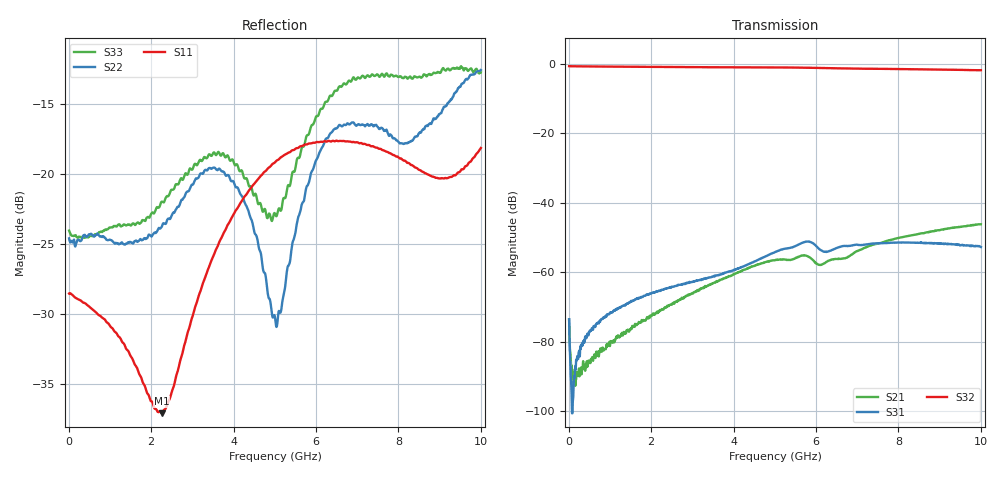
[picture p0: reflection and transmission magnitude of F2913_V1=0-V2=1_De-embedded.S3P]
! Webpage:  http://www.idt.com/
! Timing and RF Division
! 515 Groton Road, Suite 102
! Westford, MA 01886-6024
! Device:  F2913
! Description: High Isolation SP2T RF Switch
! Frequency:  0.050 -  6.000 GHz
! Package:  4x4 mm QFN Plastic Package: 20 pin
! Ports:  3 RF, 3 DC
!  Pin  1  = GND
!  Pin  2  = GND
!  Pin  3  = RF1  =  Port 1
!  Pin  4  = GND
!  Pin  5  = GND
!  Pin  6  = GND
!  Pin  7  = GND
!  Pin  8  = RFC  =  Port 3
!  Pin  9  = GND
!  Pin 10  = GND
!  Pin 11  = GND
!  Pin 12  = GND
!  Pin 13  = RF2  =  Port 2
!  Pin 14  = GND
!  Pin 15  = GND
!  Pin 16  = C2
!  Pin 17  = C1
!  Pin 18  = GND
!  Pin 19  = GND
!  Pin 20  = Vdd
! State:  RF2 Selected
! C1:  0.0 V (Logic Low)
! C2:  +3.3 V (Logic High)
! Voltage:  +3.30  Volts
! Current:  0.082 mA
! Data:  The device was measured on a F2913 evaluation board which has
!  individual transmission lines to the RF pins.  Data was collected
!  using a calibrated network analyzer.  The evaluation board was
!  de-embedded using a AFR (Keysight Technologies).
!  The reference plane is the edge of the package pin.
! Misc:
!  Action Tracker AT0430
!  WorkFront Reference Number 1053824
! Date Measured:  2018-08-23
! Date:  2018-08-24  MJV
! Note:
!  Integrated Device Technology supplies this data as a sample of measured
!  data at the package pin for this product.  Your particular data for this
!  product may vary.
!  Data was taken at 25 degrees C.
!  Integrated Device Technology reserves the right to change this data at anytime.
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# Hz S dB R 50
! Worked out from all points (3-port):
!   1000 points, 10 MHz to 10 GHz, reference 50 ohm
!   strongest paths, dB at 10 MHz, 2.51 GHz, 5.01 GHz, 7.51 GHz, 10 GHz:
!     S32: -0.7, -0.9, -1.0, -1.4, -1.8
!     S31: -73.5, -64.2, -54.2, -51.6, -52.7
!     S21: -73.6, -69.0, -56.5, -51.7, -46.2
!   lowest |S11| = -37.1 dB at 2.26 GHz (marker M1), VSWR 1.03, Z = 49.1 + j1.07 ohm
!   |S11| at or under -10 dB: start of sweep to end of sweep
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1e7  -28.51 -179.7  -73.49 -49.4  -72.94 -44.8
     -73.56 -47.5  -24.58 -1.7  -0.69 -0.3
     -73.51 -41.7  -0.67 -0.3  -24.02 -1.9
7e7  -28.57 178.7  -88.19 -88.0  -95.74 -46.9
     -86.78 -87.8  -24.80 -5.3  -0.71 -1.3
     -95.24 -20.1  -0.70 -1.3  -24.38 -3.3
3.2e8  -29.09 175.4  -88.62 -110.0  -80.77 75.1
       -88.52 -100.8  -24.64 -13.0  -0.74 -5.3
       -81.24 75.4  -0.73 -5.3  -24.53 -10.0
1.03e9  -30.93 173.3  -79.68 -121.5  -71.69 79.5
        -80.02 -122.3  -24.70 -25.3  -0.80 -16.7
        -71.52 79.7  -0.80 -16.7  -23.79 -29.1
2.26e9  -37.07 128.9  -71.01 -149.9  -65.12 80.7
        -70.57 -148.5  -23.74 -4.4  -0.89 -36.4
        -65.04 80.3  -0.90 -36.3  -21.96 -19.7
3.73e9  -24.38 88.1  -61.85 174.7  -60.40 84.9
        -62.02 174.4  -19.80 18.5  -0.99 -60.2
        -60.47 85.4  -0.99 -60.2  -18.52 -14.4
5.01e9  -19.13 105.9  -56.44 134.9  -54.15 80.1
        -56.49 135.1  -30.33 81.0  -1.02 -81.4
        -54.17 80.1  -1.03 -81.4  -22.85 -88.7
6.38e9  -17.65 121.4  -56.33 116.3  -53.64 52.2
        -56.35 116.0  -17.01 145.9  -1.26 -103.4
        -53.60 52.2  -1.26 -103.5  -14.42 -161.3
8.25e9  -19.20 117.9  -49.48 95.6  -51.45 29.9
        -49.52 96.0  -17.73 71.5  -1.52 -132.1
        -51.44 29.9  -1.51 -132.0  -13.09 -158.4
1e10  -18.13 62.7  -46.16 64.4  -52.67 7.1
      -46.16 64.3  -12.56 6.2  -1.82 -162.0
      -52.72 6.8  -1.83 -162.2  -12.72 -158.4
